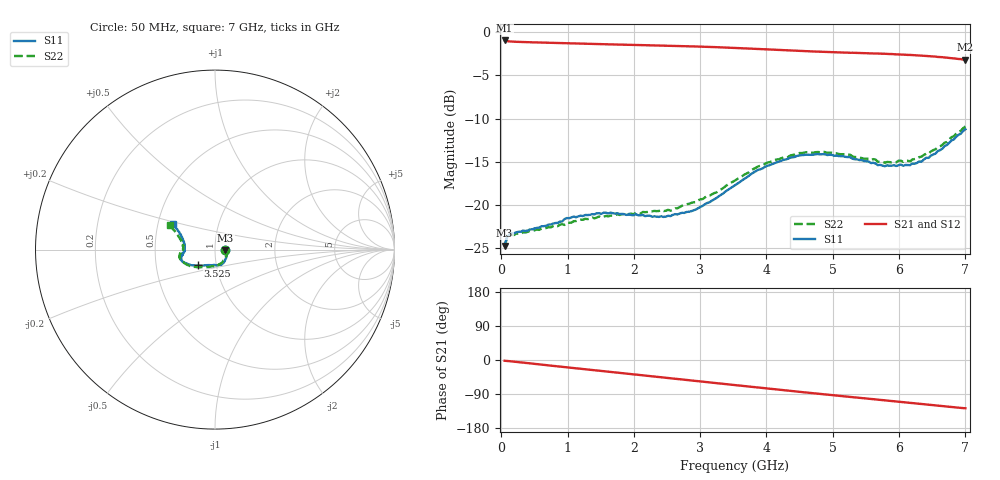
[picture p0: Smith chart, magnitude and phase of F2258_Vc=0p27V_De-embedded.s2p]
! Integrated Device Technology
! Corporate Headquarters
! 6024 Silver Creek Valley Road
! San Jose, CA 95138  USA
! Phone:  1-408-284-8200
! Toll Free:  1-800-223-1366
! Webpage:  http://www.idt.com/
! Timing and RF Division
! 515 Groton Road, Suite 102
! Westford, MA 01886-6024
! Device:  F2258
! Description: Voltage Variable RF Attenuator
! Frequency:  50.0 -  6000.00 MHz
! Package:  3x3 mm Thin QFN Plastic Package: 16 pin
! Ports:  2 RF, 2 DC
!  Pin  1  = NC
!  Pin  2  = NC
!  Pin  3  = RF2  = Port 2
!  Pin  4  = GND
!  Pin  5  = Vdd
!  Pin  6  = NC
!  Pin  7  = VCTRL
!  Pin  8  = NC
!  Pin  9  = GND
!  Pin 10  = RF1  = Port 1
!  Pin 11  = NC
!  Pin 12  = NC
!  Pin 13  = NC
!  Pin 14  = NC
!  Pin 15  = NC
!  Pin 16  = NC
! Vcntrl:  0.270 Volts
! Vdd:  +3.300 Volts
! Current:  1.080 mA
! Data:  The device was measured on a the F2258 evaluation board which has
!  individual transmission lines to the RF pins.  Data was collected
!  using a calibrated network analyzer.  The evaluation board was
!  de-embedded using a TRL calibration technique.
!  The reference plane is the edge of the package pin.
! Misc:  SN 10
!  Action Tracker AT0285
! Date Measured:  2014-12-10
! Date:  2016-01-13  MJV
! Note:
!  Integrated Device Technology supplies this data as a sample of measured
!  data at the package pin for this product.  Your particular data for this
!  product may vary.
!  Data was taken at 25 degrees C.
!  Integrated Device Technology reserves the right to change this data at anytime.
!Freq_(GHz)  S11M_(dB)  S11P_(deg)  S21M_(dB)  S21P_(deg)  S12M_(dB)  S12P_(deg)  S22M_(dB)  S22P_(deg)
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# GHz S dB R 50
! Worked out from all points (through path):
!   201 points, 50 MHz to 7 GHz, reference 50 ohm
!   highest |S21| = -0.97 dB at 50 MHz (marker M1); lowest = -3.2 dB at 7 GHz (marker M2)
!   group delay of S21, straight-line fit = 50.5 ps
!   lowest |S11| = -24.7 dB at 50 MHz (marker M3), VSWR 1.12, Z = 56.2 - j0.391 ohm
!   |S11| at or under -10 dB: start of sweep to end of sweep
!   |S22| runs from -24.7 to -10.9 dB; largest |S21 - S12| = 0.00036
!   S11 on the Smith chart (normalised r, x): 50 MHz: 1.12, -0.01; 3.525 GHz: 0.81, -0.15; 7 GHz: 0.60, +0.19
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0.05  -24.67 -3.4  -0.97 -1.9  -0.97 -1.9  -24.73 -3.1
0.08475  -23.71 -5.8  -1.04 -2.5  -1.04 -2.5  -23.80 -5.4
0.15425  -23.22 -9.1  -1.10 -3.6  -1.10 -3.6  -23.42 -9.4
0.71025  -22.24 -36.6  -1.23 -14.1  -1.23 -14.1  -22.53 -38.3
0.91875  -21.87 -46.4  -1.27 -18.0  -1.27 -18.0  -22.19 -50.0
0.98825  -21.49 -50.4  -1.28 -19.3  -1.28 -19.3  -22.04 -54.3
1.2315  -21.25 -58.6  -1.34 -23.8  -1.34 -23.8  -21.68 -63.3
1.6485  -20.86 -70.3  -1.42 -31.4  -1.42 -31.4  -21.20 -76.3
2.37825  -21.35 -91.5  -1.55 -44.8  -1.55 -44.8  -20.66 -94.0
2.552  -21.26 -97.5  -1.58 -48.0  -1.58 -48.0  -20.63 -99.3
2.93425  -20.51 -114.2  -1.67 -55.1  -1.67 -55.1  -19.64 -112.7
3.525  -17.71 -137.1  -1.83 -66.2  -1.83 -66.2  -17.15 -135.4
4.0115  -15.45 -150.9  -2.01 -75.2  -2.01 -75.2  -15.08 -150.8
4.46325  -14.30 -159.3  -2.17 -83.4  -2.17 -83.4  -14.03 -161.9
4.7065  -14.17 -162.6  -2.24 -87.7  -2.24 -87.7  -13.93 -166.2
5.15825  -14.33 -168.1  -2.37 -95.6  -2.37 -95.6  -14.11 -173.1
5.6795  -15.37 -176.3  -2.48 -104.6  -2.48 -104.6  -14.98 -179.6
5.85325  -15.44 179.5  -2.53 -107.8  -2.54 -107.8  -15.02 175.8
6.166  -15.37 171.7  -2.64 -113.4  -2.64 -113.4  -14.93 169.8
6.33975  -14.96 165.3  -2.72 -116.5  -2.73 -116.5  -14.39 165.5
6.722  -13.05 153.6  -2.96 -123.1  -2.96 -123.1  -12.68 156.4
7  -11.23 148.2  -3.20 -127.4  -3.21 -127.4  -10.90 151.5
